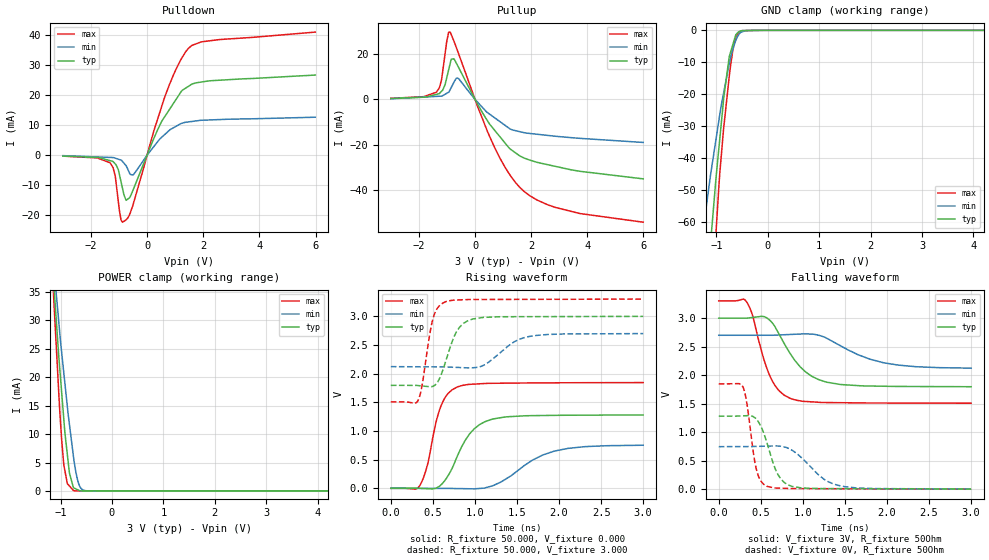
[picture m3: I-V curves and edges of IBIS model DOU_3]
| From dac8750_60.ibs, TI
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|   DOU Models
[Model] DOU_3  |3V digital 3-state output
Model_type   3-state
Polarity   Non-Inverting
Vmeas = 1.5
Vref = 1.5
Cref = 0pF
Rref = 50
|   typ   min   max
|   (nom PVT)   (Fast PVT)   (slow PVT)
|   BUFFER OUTPUT TURNED HIGH
C_comp   1.812E-12   1.294E-12   1.959E-12
|   BUFFER OUTPUT LOW
|C_comp   1.734E-12   1.226E-12   1.837E-12
|   BUFFER HIGH Z STATE
|C_comp   1.691E-12   1.087E-12   1.754E-12
| Where   nom PVT is  Nominal Process, 3.0V, 36C
|   Fast PVT is Strong Process, 3.3V, -40C
|   Slow PVT is Weak Process, 2,7V, 134C
|C_comp - from L-C Tank method, L = 1nH, peak frequency
[Voltage Range]   3   2.7   3.3
[Temperature Range]   36   134   -40
|Operating Temperature   27   125   -40
|Junction Temperature
[Pullup Reference]   3   2.7   3.3
[Pulldown Reference]   0   0   0
[Power Clamp Reference]   3   2.7   3.3
[GND Clamp Reference]   -0   0   0
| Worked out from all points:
|   slope of the pulldown table from 0 to 0.45 V, typ, clamps not added: 45.5 ohm
|   slope of the pullup table from 0 to 0.45 V, typ, clamps not added: 47 ohm
|   GND clamp passes 1 mA (typ) near -0.60 V on its own axis
|   POWER clamp passes 1 mA (typ) near -0.76 V on its own axis
|   falling waveform, V_fixture 3V, R_fixture 50Ohm: 20-80 % time 349ps typ, 543ps min, 228ps max; typ from 3 V to 1.8 V
|   rising waveform, R_fixture 50.000, V_fixture 0.000: 20-80 % time 287ps typ, 493ps min, 180ps max; typ from 0.003 V to 1.28 V
|   rising waveform, R_fixture 50.000, V_fixture 3.000: 20-80 % time 180ps typ, 309ps min, 119ps max; typ from 1.8 V to 3 V
|   falling waveform, V_fixture 0V, R_fixture 50Ohm: 20-80 % time 180ps typ, 327ps min, 107ps max; typ from 1.28 V to 0.003 V
[Pulldown]
|   Voltage   I(typ)   I(min)   I(max)
-3V       -312.6uA   -191.7uA   -346.7uA
-1.312V   -1.872mA   -787.5uA   -2.653mA
-1.137V   -2.918mA   -1.028mA   -6.928mA
-986.5mV  -6.499mA   -1.49mA    -18.51mA
-874.7mV  -11.17mA   -2.138mA   -22.35mA
-749.5mV  -15.06mA   -3.533mA   -21.58mA
-621.8mV  -14.19mA   -6.069mA   -19.77mA
-489.3mV  -11.36mA   -6.495mA   -16.15mA
606.7mV   12.49mA    6.677mA    18.75mA
1.46V     22.82mA    11.03mA    35.43mA
1.942V    24.34mA    11.6mA     37.72mA
5.991V    26.65mA    12.61mA    40.96mA
[GND Clamp]
|   Voltage   I(typ)   I(min)   I(max)
-3V       -490.7mA   -317.9mA   -695.7mA
-1.353V   -114.8mA   -73.75mA   -166.9mA
-1.196V   -82.27mA   -55mA      -117.6mA
-1.11V    -65.87mA   -44.81mA   -92.09mA
-1.036V   -51.72mA   -37.07mA   -70.54mA
-1.003V   -45.44mA   -33.61mA   -62.11mA
-934.4mV  -33.99mA   -26.37mA   -44.76mA
-861mV    -21.81mA   -19.7mA    -30.97mA
-744.5mV  -7.896mA   -9.969mA   -13.61mA
-659.6mV  -3.374mA   -4.834mA   -4.627mA
-568.8mV  -462.3uA   -1.441mA   -666uA
5.991V    0A         0A         0A
[Pullup]
|   Voltage   I(typ)   I(min)   I(max)
-3V       390uA      274.3uA    463.1uA
-1.372V   2.22mA     1.326mA    3.229mA
-1.268V   2.621mA    1.394mA    5.187mA
-1.155V   4.031mA    1.624mA    12.08mA
-1.012V   9.32mA     2.658mA    25.23mA
-881.3mV  16.04mA    4.409mA    29.64mA
-749.5mV  17.94mA    7.656mA    25.7mA
-589mV    14.18mA    9.173mA    20.29mA
665.3mV   -13.15mA   -7.83mA    -20.38mA
1.592V    -24.95mA   -14.25mA   -38.82mA
2.856V    -29.56mA   -16.27mA   -47.69mA
5.991V    -35.1mA    -19.02mA   -54.23mA
[POWER Clamp]
|   Voltage   I(typ)   I(min)   I(max)
-3V       311.6mA    246mA      408.2mA
-1.137V   37.19mA    40.08mA    34.67mA
-1.128V   35.91mA    39.11mA    32.93mA
-1.038V   24.07mA    30.07mA    17.8mA
-981.6mV  17.69mA    24.62mA    9.395mA
-942.6mV  13.27mA    21.26mA    5.135mA
-867.9mV  6.396mA    14.83mA    1.283mA
-827.6mV  3.154mA    11.73mA    874.4uA
-744.5mV  534.5uA    5.714mA    32.06uA
-643.3mV  101.4uA    1.168mA    2.644uA
-510.9mV  1.472uA    38.92uA    5.614nA
5.991V    0A         0A         0A
[Ramp]
R_load = 50
|   typ   min   max
dV/dt_r   0.766199/2.85826e-010  0.444635/4.84148e-010   1.10585/1.78901e-010
dV/dt_f   0.721171/3.46067e-010  0.345711/5.32764e-010   1.07549/2.27952e-010
[Falling Waveform]
V_fixture = 3V
V_fixture_min = 2.7V
V_fixture_max = 3.3V
R_fixture = 50Ohm
C_fixture = 0F
|   Time   V(typ)   V(min)   V(max)
0s        2.998V     2.698V     3.3V
327.4ps   2.999V     2.698V     3.293V
401.4ps   3.01V      2.698V     3.051V
521.3ps   3.028V     2.698V     2.352V
611.1ps   2.957V     2.698V     1.975V
847.9ps   2.38V      2.712V     1.594V
1.034ns   2.054V     2.723V     1.538V
1.289ns   1.874V     2.642V     1.519V
1.957ns   1.805V     2.218V     1.511V
3ns       1.796V     2.122V     1.507V
[Rising Waveform]
R_fixture = 50.000
V_fixture = 0.000
V_fixture_min = 0.000
V_fixture_max = 0.000
C_fixture = 0.000
|  time   V(typ)   V(min)   V(max)
0s        3.176mV    1.168uV    937.3uV
343.4ps   963.5uV    -286.8uV   45.3mV
437.4ps   -5.045mV   -365.7uV   420.1mV
527.4ps   -38.87uV   -441.2uV   1.09V
594.8ps   58.88mV    -497.7uV   1.432V
787.2ps   550.3mV    -3.19mV    1.766V
991.1ps   1.038V     -8.047mV   1.818V
1.211ns   1.209V     45.16mV    1.832V
1.936ns   1.273V     646.5mV    1.84V
3ns       1.28V      752mV      1.844V
[Rising Waveform]
R_fixture = 50.000
V_fixture = 3.000
V_fixture_min = 2.700
V_fixture_max = 3.300
C_fixture = 0.000
|  time   V(typ)   V(min)   V(max)
0s        1.796V     2.122V     1.507V
323ps     1.793V     2.12V      1.529V
371.1ps   1.785V     2.119V     1.793V
498.7ps   1.778V     2.119V     2.946V
562.7ps   1.868V     2.118V     3.158V
643.4ps   2.174V     2.118V     3.25V
784.1ps   2.74V      2.109V     3.284V
979.5ps   2.954V     2.103V     3.293V
1.64ns    2.993V     2.646V     3.295V
3ns       2.998V     2.698V     3.3V
[Falling Waveform]
|Gnd
V_fixture = 0V
V_fixture_min = 0V
V_fixture_max = 0V
R_fixture = 50Ohm
C_fixture = 0F
|   Time   V(typ)   V(min)   V(max)
0s        1.28V      745.7mV    1.844V
289.2ps   1.286V     747.3mV    1.789V
336.4ps   1.289V     747.6mV    1.485V
445.9ps   1.232V     750mV      358.6mV
497.4ps   1.111V     752.2mV    150.8mV
572.8ps   816.9mV    755.3mV    51.15mV
704.1ps   256.8mV    756.8mV    19.75mV
877.1ps   47.23mV    678.7mV    11.11mV
1.42ns    10.34mV    67.34mV    8.506mV
3ns       3.302mV    3.956mV    938.1uV
